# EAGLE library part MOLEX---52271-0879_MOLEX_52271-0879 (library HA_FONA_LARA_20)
MOLX-52271-0879
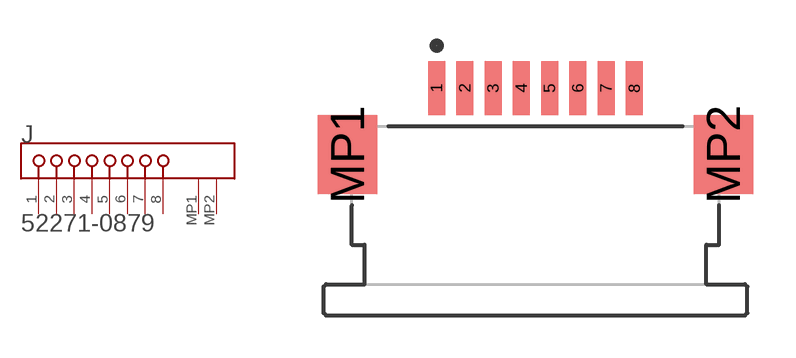
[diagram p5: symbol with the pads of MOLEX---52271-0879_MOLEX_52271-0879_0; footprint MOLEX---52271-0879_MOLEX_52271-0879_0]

Designator prefix J

## MOLEX---52271-0879_MOLEX_52271-0879MOLEX_52271-0879_0_0 (CIIVA_IDS: 605436; CIRCUITS_LOADED: 8; COMPONENT_LINK_1_DESCRIPTION: Manufacturer URL; COMPONENT_LINK_1_URL: http://www.molex.com/molex/index.jsp; COMPONENT_LINK_3_DESCRIPTION: Package Specification; COMPONENT_LINK_3_URL: http://www.molex.com/pdm_docs/sd/522710879_sd.pdf; CONTACT_POSITION: Bottom; CURRENT_MAX_PER_CONTACT: 0.5A; DATASHEET: http://www.molex.com/webdocs/datasheets/pdf/en-us/0522710879_FFC_FPC_CONNECTORS.pdf; DURABILITY_MATING_CYCLES_MAX: 30; ENTRY_ANGLE: 90degrees Angle; FOOTPRINT_VARIANT_NAME_0: Manufacturer Recommended; IMPORTED: yes; IMPORTED_FROM: vault; IMPORT_TS: 1521845783; MATED_HEIGHT: 3.00mm; MATERIAL___METAL: Phosphor Bronze; MATERIAL___PLATING_MATING: Tin-Bismuth; MATERIAL___PLATING_TERMINATION: Tin-Bismuth; MF: Molex; MOUNTING_TECHNOLOGY: Surface Mount; MPN: 52271-0879; NUMBER_OF_ROWS: 1; ORIENTATION: Right Angle; PACKAGE: 52271-0879; PACKAGE_DESCRIPTION: 8-Lead FPC Connector, Pitch 1.0 mm; PACKAGE_VERSION: Rev. B, 04/2004; PACKING: Tape and Reel; PCB_LOCATOR: No; PCB_RETENTION: Yes; PITCH___MATING_INTERFACE: 1.00mm; PITCH___TERMINATION_INTERFACE: 1.00mm; POLARIZED_TO_PCB: Yes; PREFIX: J; RELEASE_DATE: 1411372468; ROHS: Yes; STACKABLE: No; VAULT_GUID: 6E0E35AC-EB58-4C9C-8B40-B34D68BAFD49; VAULT_REVISION: B8D0B5D1-BD2E-4A74-BF2B-C0B6D1E0611E; VOLTAGE_MAX: 50V AC (RMS)/DC)  [MOLEX---52271-0879_MOLEX_52271-0879_0]
1  1  pas
2  2  pas
3  3  pas
4  4  pas
5  5  pas
6  6  pas
7  7  pas
8  8  pas
MP1  MP1  pas
MP2  MP2  pas

## Footprint MOLEX---52271-0879_MOLEX_52271-0879_0 (pad centres in mm)
MOLX-52271-0879
smd 0.6 x 1.9: 1 -3.5,1.175; 2 -2.5,1.175; 3 -1.5,1.175; 4 -0.5,1.175; 5 0.5,1.175; 6 1.5,1.175; 7 2.5,1.175; 8 3.5,1.175
smd 2.1 x 2.8: MP1 -6.65,-1.175; MP2 6.65,-1.175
